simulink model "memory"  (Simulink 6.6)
settings: Solver=ode45  StartTime=0.0  StopTime=25.0  RelTol=1e-3
undefined symbols (not defined in the file or in its folder): adlibrary2, ADM, Bit, DDRII, DRAM, Location, Lower, netlist, Width, XRC
libraries: xbsIndex_r4 x36, adlibrary2_ddr2dram5t1_1 x1, adlibrary2 x1

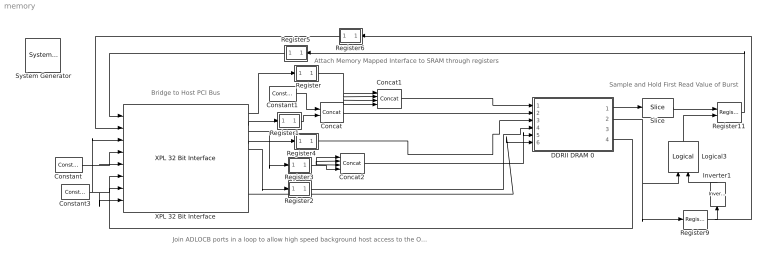
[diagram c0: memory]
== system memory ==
  note: Bridge to Host PCI Bus
  note: Attach Memory Mapped Interface to SRAM through registers
  note: Join ADLOCB ports in a loop to allow high speed background host access to the Off Chip Ram
  note: Sample and Hold First Read Value of Burst
  " System Generator" : xbsIndex_r4/ System Generator  Tag=genX  SystemSampleTime=-1  xilinxfamily=virtex5  part=xc5vlx330t  speed=-1  package=ff1738  synthesis_tool=XST  directory=./netlist  testbench=off  simulink_period=1  sysclk_period=6  incr_netlist=off  trim_vbits=Everywhere in SubSystem  dbl_ovrd=According to Block Masks  core_generation=According to Block Masks  run_coregen=off  deprecated_control=off  eval_field=0  block_type=sysgen
  Concat : xbsIndex_r4/Concat  num_inputs=2  dbl_ovrd=off  block_type=concat
  Concat1 : xbsIndex_r4/Concat  num_inputs=4  dbl_ovrd=off  block_type=concat
  Concat2 : xbsIndex_r4/Concat  num_inputs=4  dbl_ovrd=off  block_type=concat
  Constant : xbsIndex_r4/Constant  arith_type=Boolean  const=0  n_bits=1  bin_pt=0  explicit_period=on  period=1  equ=P=C  opselect=C  inp2=PCIN>>17  opr=+  inp1=P  carry=CIN  dbl_ovrd=off  block_type=constant
  Constant1 : xbsIndex_r4/Constant  arith_type=Unsigned  const=0  n_bits=12  bin_pt=0  explicit_period=on  period=1  equ=P=C  opselect=C  inp2=PCIN>>17  opr=+  inp1=P  carry=CIN  dbl_ovrd=off  block_type=constant
  Constant3 : xbsIndex_r4/Constant  arith_type=Unsigned  const=0  n_bits=32  bin_pt=0  explicit_period=on  period=1  equ=P=C  opselect=C  inp2=PCIN>>17  opr=+  inp1=P  carry=CIN  dbl_ovrd=off  block_type=constant
  DDRII DRAM 0 : Subsystem  AncestorBlock=adlibrary2/ADM-XRC-5T2/DDRII DRAM 0  mask{rate=1}
      mask prompts: rate "Simulink Clock Period"
  Inverter1 : xbsIndex_r4/Inverter  Orientation=up  en=off  latency=0  dbl_ovrd=off  block_type=inv
  Logical3 : xbsIndex_r4/Logical  Orientation=up  logical_function=AND  inputs=2  en=off  latency=0  precision=Full  arith_type=Unsigned  n_bits=8  bin_pt=2  align_bp=on  dbl_ovrd=off  block_type=logical
  Register : Subsystem
  Register1 : Subsystem
  Register11 : xbsIndex_r4/Register  init=0  rst=off  en=on  dbl_ovrd=off  block_type=register
  Register2 : Subsystem
  Register3 : Subsystem
  Register4 : Subsystem
  Register5 : Subsystem  Orientation=left
  Register6 : Subsystem  Orientation=left
  Register9 : xbsIndex_r4/Register  init=0  rst=off  en=off  dbl_ovrd=off  block_type=register
  Slice : xbsIndex_r4/Slice  nbits=32  boolean_output=off  mode=Lower Bit Location + Width  bit1=0  base1=MSB of Input  bit0=0  base0=LSB of Input  dbl_ovrd=off  block_type=slice
  XPL 32 Bit Interface : adlibrary2/ADM-XPL/XPL 32 Bit Interface  SystemSampleTime=-1  program='slave_write 0x0 0x1234;slave_read 0x0'  clock_ratio=1.5  sstep_clk_sel_default=0
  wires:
  Constant/1 -> XPL 32 Bit Interface/4, XPL 32 Bit Interface/5
  Constant3/1 -> XPL 32 Bit Interface/8, XPL 32 Bit Interface/6, XPL 32 Bit Interface/3
  XPL 32 Bit Interface/5 -> Register2/1(in0)
  XPL 32 Bit Interface/2 -> Register1/1(in0)
  XPL 32 Bit Interface/1 -> Register/1(in0)
  Register/1(out0) -> Concat1/1, Concat1/2, Concat1/3, Concat1/4
  Register4/1(out0) -> DDRII DRAM 0/3(w)
  Constant1/1 -> Concat/1
  Register1/1(out0) -> Concat/2
  Register5/1(out0) -> XPL 32 Bit Interface/1
  Register6/1(out0) -> XPL 32 Bit Interface/2
  Register3/1(out0) -> Concat2/1, Concat2/2, Concat2/3, Concat2/4
  XPL 32 Bit Interface/4 -> Register4/1(in0)
  XPL 32 Bit Interface/3 -> Register3/1(in0)
  DDRII DRAM 0/4(adlocb_out) -> XPL 32 Bit Interface/7
  XPL 32 Bit Interface/10 -> DDRII DRAM 0/6(adlocb_in)
  Register2/1(out0) -> DDRII DRAM 0/4(r)
  DDRII DRAM 0/1(q) -> Slice/1
  Slice/1 -> Register11/1
  Logical3/1 -> Register11/2
  Inverter1/1 -> Logical3/2
  DDRII DRAM 0/2(qv) -> Register9/1, Logical3/1
  Register9/1 -> Inverter1/1, Register6/1(in0)
  Register11/1 -> Register5/1(in0)
  Concat2/1 -> DDRII DRAM 0/5(be)
  Concat1/1 -> DDRII DRAM 0/1(d)
  Concat/1 -> DDRII DRAM 0/2(a)

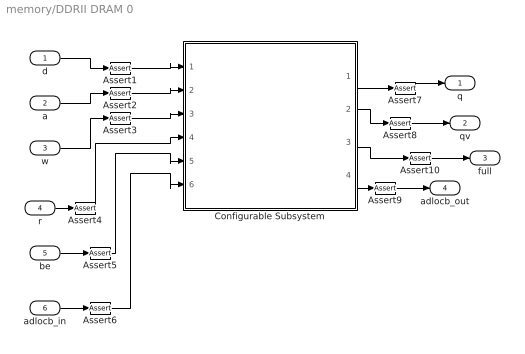
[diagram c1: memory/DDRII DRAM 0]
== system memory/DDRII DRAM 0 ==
  d : Inport
  a : Inport  Port=2
  w : Inport  Port=3
  r : Inport  Port=4
  be : Inport  Port=5
  adlocb_in : Inport  Port=6
  Assert{1..10} (10 alike) : xbsIndex_r4/Assert  assert_type=off  type_source=Explicitly  arith_type="Signed  (2's comp)"  n_bits=16  bin_pt=14  assert_rate=on  rate_source=Explicitly  period=ad_get_simulink_period  output_port=on  block_type=assert
  Configurable Subsystem : Subsystem  Tag=configX  BlockChoice=DDRII DRAM Simulation
  q : Outport
  qv : Outport  Port=2
  full : Outport  Port=3
  adlocb_out : Outport  Port=4
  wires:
  Configurable Subsystem/3(full) -> Assert10/1
  Assert10/1 -> full/1
  Configurable Subsystem/1(q) -> Assert7/1
  d/1 -> Assert1/1
  a/1 -> Assert2/1
  w/1 -> Assert3/1
  r/1 -> Assert4/1
  be/1 -> Assert5/1
  adlocb_in/1 -> Assert6/1
  Configurable Subsystem/4(adlocb_out) -> Assert9/1
  Configurable Subsystem/2(qv) -> Assert8/1
  Assert1/1 -> Configurable Subsystem/1(d)
  Assert2/1 -> Configurable Subsystem/2(a)
  Assert3/1 -> Configurable Subsystem/3(w)
  Assert4/1 -> Configurable Subsystem/4(r)
  Assert5/1 -> Configurable Subsystem/5(be)
  Assert6/1 -> Configurable Subsystem/6(adlocb_in)
  Assert7/1 -> q/1
  Assert8/1 -> qv/1
  Assert9/1 -> adlocb_out/1

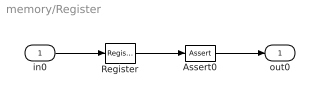
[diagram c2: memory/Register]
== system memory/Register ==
  in0 : Inport
  Assert0 : xbsIndex_r4/Assert  assert_type=off  type_source=Explicitly  arith_type="Signed  (2's comp)"  n_bits=16  bin_pt=14  assert_rate=on  rate_source=Explicitly  period=1  output_port=on  block_type=assert
  Register : xbsIndex_r4/Register  init=0  rst=off  en=off  dbl_ovrd=off  block_type=register
  out0 : Outport
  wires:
  in0/1 -> Register/1
  Register/1 -> Assert0/1
  Assert0/1 -> out0/1

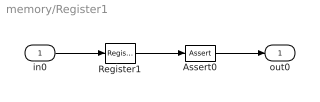
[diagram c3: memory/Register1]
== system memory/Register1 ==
  in0 : Inport
  Assert0 : xbsIndex_r4/Assert  assert_type=off  type_source=Explicitly  arith_type="Signed  (2's comp)"  n_bits=16  bin_pt=14  assert_rate=on  rate_source=Explicitly  period=1  output_port=on  block_type=assert
  Register1 : xbsIndex_r4/Register  init=0  rst=off  en=off  dbl_ovrd=off  block_type=register
  out0 : Outport
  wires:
  in0/1 -> Register1/1
  Register1/1 -> Assert0/1
  Assert0/1 -> out0/1

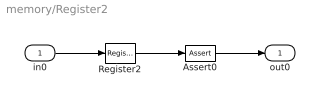
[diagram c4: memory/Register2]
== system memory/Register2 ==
  in0 : Inport
  Assert0 : xbsIndex_r4/Assert  assert_type=off  type_source=Explicitly  arith_type="Signed  (2's comp)"  n_bits=16  bin_pt=14  assert_rate=on  rate_source=Explicitly  period=1  output_port=on  block_type=assert
  Register2 : xbsIndex_r4/Register  init=0  rst=off  en=off  dbl_ovrd=off  block_type=register
  out0 : Outport
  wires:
  in0/1 -> Register2/1
  Register2/1 -> Assert0/1
  Assert0/1 -> out0/1

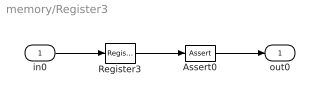
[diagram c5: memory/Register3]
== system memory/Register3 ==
  in0 : Inport
  Assert0 : xbsIndex_r4/Assert  assert_type=off  type_source=Explicitly  arith_type="Signed  (2's comp)"  n_bits=16  bin_pt=14  assert_rate=on  rate_source=Explicitly  period=1  output_port=on  block_type=assert
  Register3 : xbsIndex_r4/Register  init=0  rst=off  en=off  dbl_ovrd=off  block_type=register
  out0 : Outport
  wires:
  in0/1 -> Register3/1
  Register3/1 -> Assert0/1
  Assert0/1 -> out0/1

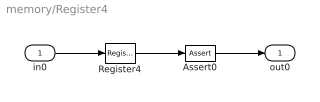
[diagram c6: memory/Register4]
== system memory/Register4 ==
  in0 : Inport
  Assert0 : xbsIndex_r4/Assert  assert_type=off  type_source=Explicitly  arith_type="Signed  (2's comp)"  n_bits=16  bin_pt=14  assert_rate=on  rate_source=Explicitly  period=1  output_port=on  block_type=assert
  Register4 : xbsIndex_r4/Register  init=0  rst=off  en=off  dbl_ovrd=off  block_type=register
  out0 : Outport
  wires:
  in0/1 -> Register4/1
  Register4/1 -> Assert0/1
  Assert0/1 -> out0/1

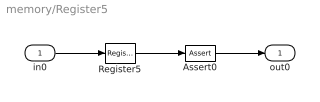
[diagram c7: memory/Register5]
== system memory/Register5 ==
  in0 : Inport
  Assert0 : xbsIndex_r4/Assert  assert_type=off  type_source=Explicitly  arith_type="Signed  (2's comp)"  n_bits=16  bin_pt=14  assert_rate=on  rate_source=Explicitly  period=1  output_port=on  block_type=assert
  Register5 : xbsIndex_r4/Register  init=0  rst=off  en=off  dbl_ovrd=off  block_type=register
  out0 : Outport
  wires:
  in0/1 -> Register5/1
  Register5/1 -> Assert0/1
  Assert0/1 -> out0/1

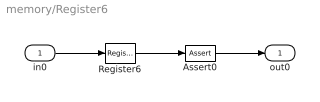
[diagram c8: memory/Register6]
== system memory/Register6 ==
  in0 : Inport
  Assert0 : xbsIndex_r4/Assert  assert_type=off  type_source=Explicitly  arith_type="Signed  (2's comp)"  n_bits=16  bin_pt=14  assert_rate=on  rate_source=Explicitly  period=1  output_port=on  block_type=assert
  Register6 : xbsIndex_r4/Register  init=0  rst=off  en=off  dbl_ovrd=off  block_type=register
  out0 : Outport
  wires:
  in0/1 -> Register6/1
  Register6/1 -> Assert0/1
  Assert0/1 -> out0/1

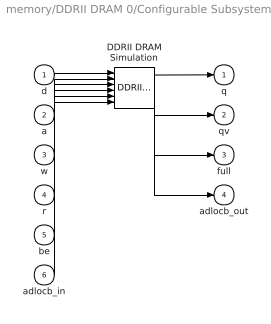
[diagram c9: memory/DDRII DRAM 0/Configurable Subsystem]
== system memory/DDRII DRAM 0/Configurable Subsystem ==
  d : Inport
  a : Inport  Port=2
  w : Inport  Port=3
  r : Inport  Port=4
  be : Inport  Port=5
  adlocb_in : Inport  Port=6
  DDRII DRAM Simulation : adlibrary2_ddr2dram5t1_1/DDRII DRAM Simulation  SystemSampleTime=-1
  q : Outport
  qv : Outport  Port=2
  full : Outport  Port=3
  adlocb_out : Outport  Port=4
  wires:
  d/1 -> DDRII DRAM Simulation/1
  a/1 -> DDRII DRAM Simulation/2
  w/1 -> DDRII DRAM Simulation/3
  r/1 -> DDRII DRAM Simulation/4
  be/1 -> DDRII DRAM Simulation/5
  adlocb_in/1 -> DDRII DRAM Simulation/6
  DDRII DRAM Simulation/1 -> q/1
  DDRII DRAM Simulation/2 -> qv/1
  DDRII DRAM Simulation/3 -> full/1
  DDRII DRAM Simulation/4 -> adlocb_out/1
